| IBIS file was generated by Viper version: 2022.03.25
[IBIS Ver]   4.2
[Comment Char]   |_char
[File Name]   n9xx_150mhz_100hlqfp_14x14_p02g.ibs
[File Rev]   1.0
[Date]   Mon Apr  4 13:26:27 2022
[Source]   NXP Viper 2022.03.25
[Notes]
[Disclaimer] IMPORTANT NOTICE
  This information is provided on an AS IS basis and without warranty.
  IN NO EVENT SHALL NXP BE LIABLE FOR INCIDENTAL OR CONSEQUENTIAL
  DAMAGES ARISING FROM USE OF THIS INFORMATION. THIS DISCLAIMER OF
  WARRANTY EXTENDS TO THE USER OF THE INFORMATION, AND TO THEIR CUSTOMERS
  OR USERS OF PRODUCTS  AND IS IN LIEU OF ALL WARRANTIES WHETHER EXPRESS,
  IMPLIED, OR STATUTORY, INCLUDING IMPLIED WARRANTIES OF MERCHANTABILITY
  OR FITNESS FOR PARTICULAR PURPOSE.
  NXP does not represent or warrant that the information furnished
  hereunder is free of infringement of any third party patents,
  copyrights, trade secrets, or other intellectual property rights.
  NXP does not represent or warrant that the information is free of
  defect, or that it meets any particular standard, requirements or need
  of the user of the infomation or their customers.
  NXP reserves the right to change the information in this file
  without notice.
   http://www.nxp.com
[Copyright]   (C) Copyright NXP 2004 - 2022, All Rights Reserved.
|   MCXN_100HLQFP_14x14_N9XX
[Component]   MCXN_100HLQFP_14x14_N9XX
[Manufacturer]   NXP
[Package]
| variable   typ   min   max
R_pkg   0.23129   0.12177   0.27328
L_pkg   4.788e-09   3.815e-09   5.696e-09
C_pkg   3.794e-13   3.182e-13   7.043e-13
[Pin] signal_name   model_name   R_pin   L_pin   C_pin
1   P1_8   a_ip_io_3v_3p3v   0.25423   5.614e-09 4.032e-13
2   P1_9   a_ip_io_3v_3p3v   0.24672   5.246e-09 3.972e-13
3   P1_10   a_ip_io_3v_3p3v   0.24265   5.154e-09 3.883e-13
4   P1_11   a_ip_io_3v_3p3v   0.23836   5.083e-09 3.818e-13
5   P1_12   a_ip_io_3v_3p3v   0.23426   4.951e-09 3.769e-13
6   P1_13   a_ip_io_3v_3p3v   0.2353   4.835e-09 3.729e-13
7   P1_14   a_ip_io_3v_3p3v   0.2403   4.758e-09 3.682e-13
8   P1_15   a_ip_io_3v_3p3v   0.25157   4.669e-09 3.655e-13
9   RESET_B   a_ip_io_3v_3p3v   0.24167   4.709e-09 3.458e-13
10   P1_30   a_ip_io_3v_3p3v   0.2458   4.703e-09 3.510e-13
11   P1_31   a_ip_io_3v_3p3v   0.2572   4.600e-09 3.513e-13
12   VDD_CORE   POWER   NA   NA   NA
13   VDD   POWER   NA   NA   NA
14   P2_0   NC   0.27071   4.771e-09 3.447e-13
15   P2_1   a_ip_io_3v_3p3v   0.25126   4.722e-09 3.490e-13
16   P2_2   a_ip_io_3v_3p3v   0.24437   4.717e-09 3.546e-13
17   P2_3   a_ip_io_3v_3p3v   0.24352   4.712e-09 3.617e-13
18   P2_4   a_ip_io_3v_3p3v   0.24721   4.785e-09 3.684e-13
19   P2_5   a_ip_io_3v_3p3v   0.25684   4.768e-09 3.762e-13
20   P2_6   a_ip_io_3v_3p3v   0.25449   4.963e-09 3.790e-13
21   P2_7   a_ip_io_3v_3p3v   0.25831   5.064e-09 3.849e-13
22   P4_0   a_ip_io_3v_3p3v   0.15187   4.592e-09 4.366e-13
23   P4_1   a_ip_io_3v_3p3v   0.15584   4.720e-09 4.572e-13
24   P4_2   a_ip_io_3v_3p3v   0.24701   5.327e-09 4.019e-13
25   P4_3   a_ip_io_3v_3p3v   0.25004   5.370e-09 4.035e-13
26   P4_4   a_ip_io_3v_3p3v   0.16172   5.017e-09 4.680e-13
27   P4_5   a_ip_io_3v_3p3v   0.16022   4.810e-09 4.695e-13
28   P4_6   a_ip_io_3v_3p3v   0.16313   4.664e-09 4.591e-13
29   P4_7   a_ip_io_3v_3p3v   0.12458   4.127e-09 5.115e-13
30   VDD_ANA   POWER   NA   NA   NA
31   VREFH   POWER   0.14876   4.210e-09 4.282e-13
32   VREFL   GND   0.22491   4.419e-09 3.580e-13
33   VSS_P4   GND   NA   NA   NA
34   VDD_P4   POWER   NA   NA   NA
35   P4_12   a_ip_io_3v_3p3v   0.22844   4.359e-09 3.397e-13
36   P4_13   a_ip_io_3v_3p3v   0.14745   4.108e-09 3.875e-13
37   P4_15   a_ip_io_3v_3p3v   0.24012   4.708e-09 3.182e-13
38   P4_16   NC   0.24983   4.781e-09 3.254e-13
39   P4_17   a_ip_io_3v_3p3v   0.15737   4.280e-09 3.837e-13
40   P4_19   a_ip_io_3v_3p3v   0.23221   4.583e-09 3.317e-13
41   P4_20   a_ip_io_3v_3p3v   0.2327   4.602e-09 3.454e-13
42   P4_21   a_ip_io_3v_3p3v   0.146   4.143e-09 4.131e-13
43   P4_23   a_ip_io_3v_3p3v   0.23703   4.568e-09 3.483e-13
44   VDD_USB   POWER   NA   NA   NA
45   USB0_DM   NC   0.22284   4.369e-09 3.625e-13
46   USB0_DP   NC   0.23027   4.424e-09 3.739e-13
47   VDD_BAT   POWER   NA   NA   NA
48   P5_0   a_ip_io_3v_1p8v   0.23912   4.867e-09 3.839e-13
49   P5_1   a_ip_io_3v_1p8v   0.23955   5.024e-09 3.974e-13
50   P5_2   a_ip_io_3v_1p8v   0.24843   5.356e-09 4.045e-13
51   P5_3   a_ip_io_3v_1p8v   0.24798   5.176e-09 3.979e-13
52   VSS_DCDC   GND   NA   NA   NA
53   DCDC_LX   NC   0.12177   3.815e-09 7.043e-13
54   VDD_DCDC   POWER   NA   NA   NA
55   VDD_SYS   POWER   NA   NA   NA
56   P3_21   a_ip_io_3v_1p8v   0.26939   4.870e-09 3.973e-13
57   P3_20   a_ip_io_3v_1p8v   0.26266   4.731e-09 3.853e-13
58   VDD_CORE   POWER   NA   NA   NA
59   VDD_P3   POWER   NA   NA   NA
60   P3_17   a_ip_io_3v_1p8v   0.26691   4.809e-09 3.713e-13
61   P3_16   a_ip_io_3v_1p8v   0.26293   4.844e-09 3.649e-13
62   P3_15   a_ip_io_3v_1p8v   0.26865   4.990e-09 3.514e-13
63   P3_14   a_ip_io_3v_1p8v   0.27328   5.070e-09 3.477e-13
64   P3_13   a_ip_io_3v_1p8v   0.26472   4.956e-09 3.441e-13
65   P3_12   a_ip_io_3v_1p8v   0.25587   4.669e-09 3.484e-13
66   VDD_P3   POWER   NA   NA   NA
67   P3_11   a_ip_io_3v_1p8v   0.24302   4.496e-09 3.614e-13
68   P3_10   a_ip_io_3v_1p8v   0.23776   4.655e-09 3.630e-13
69   P3_9   a_ip_io_3v_1p8v   0.23969   4.796e-09 3.688e-13
70   P3_8   a_ip_io_3v_1p8v   0.242   4.857e-09 3.786e-13
71   P3_7   a_ip_io_3v_1p8v   0.24897   4.983e-09 3.880e-13
72   P3_6   a_ip_io_3v_1p8v   0.26422   4.985e-09 4.023e-13
73   VDD_P3   POWER   NA   NA   NA
74   P3_1   a_ip_io_3v_1p8v   0.25078   5.206e-09 3.982e-13
75   P3_0   a_ip_io_3v_1p8v   0.25659   5.400e-09 4.078e-13
76   P0_0   a_ip_io_3v_3p3v   0.26287   5.696e-09 4.116e-13
77   P0_1   a_ip_io_3v_3p3v   0.25446   5.469e-09 4.061e-13
78   P0_2   a_ip_io_3v_3p3v   0.23999   5.036e-09 3.921e-13
79   P0_3   a_ip_io_3v_3p3v   0.22875   4.809e-09 3.803e-13
80   P0_4   a_ip_io_3v_3p3v   0.22017   4.637e-09 3.693e-13
81   P0_5   a_ip_io_3v_3p3v   0.21763   4.557e-09 3.590e-13
82   P0_6   a_ip_io_3v_3p3v   0.21829   4.539e-09 3.430e-13
83   VDD   POWER   NA   NA   NA
84   P0_16   a_ip_io_3v_3p3v   0.23726   4.587e-09 3.470e-13
85   P0_17   a_ip_io_3v_3p3v   0.23427   4.622e-09 3.441e-13
86   P0_18   a_ip_io_3v_3p3v   0.23551   4.675e-09 3.359e-13
87   P0_19   a_ip_io_3v_3p3v   0.24397   4.807e-09 3.254e-13
88   P0_20   a_ip_io_3v_3p3v   0.25138   4.901e-09 3.222e-13
89   P0_21   a_ip_io_3v_3p3v   0.24426   4.870e-09 3.218e-13
90   P0_22   a_ip_io_3v_3p3v   0.23502   4.662e-09 3.318e-13
91   P0_23   a_ip_io_3v_3p3v   0.2362   4.512e-09 3.360e-13
92   P1_0   a_ip_io_3v_3p3v   0.22164   4.521e-09 3.323e-13
93   P1_1   a_ip_io_3v_3p3v   0.21839   4.499e-09 3.437e-13
94   P1_2   a_ip_io_3v_3p3v   0.22062   4.551e-09 3.502e-13
95   P1_3   a_ip_io_3v_3p3v   0.22417   4.511e-09 3.610e-13
96   VDD   POWER   NA   NA   NA
97   P1_4   a_ip_io_3v_3p3v   0.2327   4.698e-09 3.737e-13
98   P1_5   a_ip_io_3v_3p3v   0.23692   5.056e-09 3.809e-13
99   P1_6   a_ip_io_3v_3p3v   0.23798   5.153e-09 3.940e-13
100   P1_7   a_ip_io_3v_3p3v   0.24452   5.277e-09 3.999e-13
101   VSS   GND   NA   NA   NA
[Pin Mapping]   pulldown_ref   pullup_ref
1   NC   NC
2   NC   NC
3   NC   NC
4   NC   NC
5   NC   NC
6   NC   NC
7   NC   NC
8   NC   NC
9   NC   NC
10   NC   NC
11   NC   NC
12   NC   VDD_CORE
13   NC   VDD
14   NC   NC
15   NC   NC
16   NC   NC
17   NC   NC
18   NC   NC
19   NC   NC
20   NC   NC
21   NC   NC
22   NC   NC
23   NC   NC
24   NC   NC
25   NC   NC
26   NC   NC
27   NC   NC
28   NC   NC
29   NC   NC
30   NC   VDD_ANA
31   NC   VREFH
32   VREFL   NC
33   VSS_P4   NC
34   NC   VDD_P4
35   NC   NC
36   NC   NC
37   NC   NC
38   NC   NC
39   NC   NC
40   NC   NC
41   NC   NC
42   NC   NC
43   NC   NC
44   NC   VDD_USB
45   NC   NC
46   NC   NC
47   NC   VDD_BAT
48   NC   NC
49   NC   NC
50   NC   NC
51   NC   NC
52   VSS_DCDC   NC
53   NC   NC
54   NC   VDD_DCDC
55   NC   VDD_SYS
56   NC   NC
57   NC   NC
58   NC   VDD_CORE
59   NC   VDD_P3
60   NC   NC
61   NC   NC
62   NC   NC
63   NC   NC
64   NC   NC
65   NC   NC
66   NC   VDD_P3
67   NC   NC
68   NC   NC
69   NC   NC
70   NC   NC
71   NC   NC
72   NC   NC
73   NC   VDD_P3
74   NC   NC
75   NC   NC
76   NC   NC
77   NC   NC
78   NC   NC
79   NC   NC
80   NC   NC
81   NC   NC
82   NC   NC
83   NC   VDD
84   NC   NC
85   NC   NC
86   NC   NC
87   NC   NC
88   NC   NC
89   NC   NC
90   NC   NC
91   NC   NC
92   NC   NC
93   NC   NC
94   NC   NC
95   NC   NC
96   NC   VDD
97   NC   NC
98   NC   NC
99   NC   NC
100   NC   NC
101   VSS   NC
|*   Model Selector   *
[Model Selector] a_ip_io_3v_1p8v
p_io_25mhz_ds0_sr0_1p8v_mio   dse=0 sre=0 25mhz
p_io_25mhz_ds0_sr1_1p8v_mio   dse=0 sre=1 25mhz
p_io_25mhz_ds1_sr0_1p8v_mio   dse=1 sre=0 25mhz
p_io_25mhz_ds1_sr1_1p8v_mio   dse=1 sre=1 25mhz
p_io_25mhz_r40_ds0_sr0_1p8v_mio   dse=0 sre=0 25mhz_r40
p_io_25mhz_r40_ds0_sr1_1p8v_mio   dse=0 sre=1 25mhz_r40
p_io_25mhz_r40_ds1_sr0_1p8v_mio   dse=1 sre=0 25mhz_r40
p_io_25mhz_r40_ds1_sr1_1p8v_mio   dse=1 sre=1 25mhz_r40
p_io_50mhz_ds0_sr0_1p8v_mio   dse=0 sre=0 50mhz
p_io_50mhz_ds0_sr1_1p8v_mio   dse=0 sre=1 50mhz
p_io_50mhz_ds1_sr0_1p8v_mio   dse=1 sre=0 50mhz
p_io_50mhz_ds1_sr1_1p8v_mio   dse=1 sre=1 50mhz
p_io_25mhz_cap_ds0_sr0_1p8v_mio   dse=0 sre=0 25mhz_cap
p_io_25mhz_cap_ds0_sr1_1p8v_mio   dse=0 sre=1 25mhz_cap
p_io_25mhz_cap_ds1_sr0_1p8v_mio   dse=1 sre=0 25mhz_cap
p_io_25mhz_cap_ds1_sr1_1p8v_mio   dse=1 sre=1 25mhz_cap
p_io_25mhz_2mux_ds0_sr0_1p8v_mio   dse=0 sre=0 25mhz_2mux
p_io_25mhz_2mux_ds0_sr1_1p8v_mio   dse=0 sre=1 25mhz_2mux
p_io_25mhz_2mux_ds1_sr0_1p8v_mio   dse=1 sre=0 25mhz_2mux
p_io_25mhz_2mux_ds1_sr1_1p8v_mio   dse=1 sre=1 25mhz_2mux
p_io_100mhz_ds0_sr0_1p8v_mio   dse=0 sre=0 100mhz
p_io_100mhz_ds0_sr1_1p8v_mio   dse=0 sre=1 100mhz
p_io_100mhz_ds1_sr0_1p8v_mio   dse=1 sre=0 100mhz
p_io_100mhz_ds1_sr1_1p8v_mio   dse=1 sre=1 100mhz
p_io_100mhz_weftd_ds0_sr0_1p8v_mio   dse=0 sre=0 100mhz
p_io_100mhz_weftd_ds0_sr1_1p8v_mio   dse=0 sre=1 100mhz
p_io_100mhz_weftd_ds1_sr0_1p8v_mio   dse=1 sre=0 100mhz
p_io_100mhz_weftd_ds1_sr1_1p8v_mio   dse=1 sre=1 100mhz
p_io_i2c_ds00_ds10_sr0_1p8v_mio   dse0=0 dse1=0 sre=0 i2c
p_io_i2c_ds00_ds10_sr1_1p8v_mio   dse0=0 dse1=0 sre=1 i2c
p_io_i2c_ds00_ds11_sr0_1p8v_mio   dse0=0 dse1=1 sre=0 i2c
p_io_i2c_ds00_ds11_sr1_1p8v_mio   dse0=0 dse1=1 sre=1 i2c
p_io_i2c_ds01_ds10_sr0_1p8v_mio   dse0=1 dse1=0 sre=0 i2c
p_io_i2c_ds01_ds10_sr1_1p8v_mio   dse0=1 dse1=0 sre=1 i2c
p_io_i2c_ds01_ds11_sr0_1p8v_mio   dse0=1 dse1=1 sre=0 i2c
p_io_i2c_ds01_ds11_sr1_1p8v_mio   dse0=1 dse1=1 sre=1 i2c
p_io_i2c_i2c1_1p8v_mio   ipp_i2c_lv=1 i2c
p_io_i2cfmp_ds00_ds10_sr0_1p8v_mio   dse0=0 dse1=0 sre=0 i2cfmp
p_io_i2cfmp_ds00_ds10_sr1_1p8v_mio   dse0=0 dse1=0 sre=1 i2cfmp
p_io_i2cfmp_ds00_ds11_sr0_1p8v_mio   dse0=0 dse1=1 sre=0 i2cfmp
p_io_i2cfmp_ds00_ds11_sr1_1p8v_mio   dse0=0 dse1=1 sre=1 i2cfmp
p_io_i2cfmp_ds01_ds10_sr0_1p8v_mio   dse0=1 dse1=0 sre=0 i2cfmp
p_io_i2cfmp_ds01_ds10_sr1_1p8v_mio   dse0=1 dse1=0 sre=1 i2cfmp
p_io_i2cfmp_ds01_ds11_sr0_1p8v_mio   dse0=1 dse1=1 sre=0 i2cfmp
p_io_i2cfmp_ds01_ds11_sr1_1p8v_mio   dse0=1 dse1=1 sre=1 i2cfmp
p_io_i2cfmp_i2c1_1p8v_mio   ipp_i2c_lv=1 i2cfmp
p_io_rst_1p8v_mio   rst
p_io_rst_rx1p8v_1p8v_mio   rst
p_io_aon_1p8v_mio   rst
[Model Selector] a_ip_io_3v_3p3v
p_io_25mhz_ds0_sr0_3p3v_mio   dse=0 sre=0 25mhz
p_io_25mhz_ds0_sr1_3p3v_mio   dse=0 sre=1 25mhz
p_io_25mhz_ds1_sr0_3p3v_mio   dse=1 sre=0 25mhz
p_io_25mhz_ds1_sr1_3p3v_mio   dse=1 sre=1 25mhz
p_io_25mhz_r40_ds0_sr0_3p3v_mio   dse=0 sre=0 25mhz_r40
p_io_25mhz_r40_ds0_sr1_3p3v_mio   dse=0 sre=1 25mhz_r40
p_io_25mhz_r40_ds1_sr0_3p3v_mio   dse=1 sre=0 25mhz_r40
p_io_25mhz_r40_ds1_sr1_3p3v_mio   dse=1 sre=1 25mhz_r40
p_io_50mhz_ds0_sr0_3p3v_mio   dse=0 sre=0 50mhz
p_io_50mhz_ds0_sr1_3p3v_mio   dse=0 sre=1 50mhz
p_io_50mhz_ds1_sr0_3p3v_mio   dse=1 sre=0 50mhz
p_io_50mhz_ds1_sr1_3p3v_mio   dse=1 sre=1 50mhz
p_io_25mhz_cap_ds0_sr0_3p3v_mio   dse=0 sre=0 25mhz_cap
p_io_25mhz_cap_ds0_sr1_3p3v_mio   dse=0 sre=1 25mhz_cap
p_io_25mhz_cap_ds1_sr0_3p3v_mio   dse=1 sre=0 25mhz_cap
p_io_25mhz_cap_ds1_sr1_3p3v_mio   dse=1 sre=1 25mhz_cap
p_io_25mhz_2mux_ds0_sr0_3p3v_mio   dse=0 sre=0 25mhz_2mux
p_io_25mhz_2mux_ds0_sr1_3p3v_mio   dse=0 sre=1 25mhz_2mux
p_io_25mhz_2mux_ds1_sr0_3p3v_mio   dse=1 sre=0 25mhz_2mux
p_io_25mhz_2mux_ds1_sr1_3p3v_mio   dse=1 sre=1 25mhz_2mux
p_io_100mhz_ds0_sr0_3p3v_mio   dse=0 sre=0 100mhz
p_io_100mhz_ds0_sr1_3p3v_mio   dse=0 sre=1 100mhz
p_io_100mhz_ds1_sr0_3p3v_mio   dse=1 sre=0 100mhz
p_io_100mhz_ds1_sr1_3p3v_mio   dse=1 sre=1 100mhz
p_io_100mhz_weftd_ds0_sr0_3p3v_mio   dse=0 sre=0 100mhz
p_io_100mhz_weftd_ds0_sr1_3p3v_mio   dse=0 sre=1 100mhz
p_io_100mhz_weftd_ds1_sr0_3p3v_mio   dse=1 sre=0 100mhz
p_io_100mhz_weftd_ds1_sr1_3p3v_mio   dse=1 sre=1 100mhz
p_io_i2c_ds00_ds10_sr0_3p3v_mio   dse0=0 dse1=0 sre=0 i2c
p_io_i2c_ds00_ds10_sr1_3p3v_mio   dse0=0 dse1=0 sre=1 i2c
p_io_i2c_ds00_ds11_sr0_3p3v_mio   dse0=0 dse1=1 sre=0 i2c
p_io_i2c_ds00_ds11_sr1_3p3v_mio   dse0=0 dse1=1 sre=1 i2c
p_io_i2c_ds01_ds10_sr0_3p3v_mio   dse0=1 dse1=0 sre=0 i2c
p_io_i2c_ds01_ds10_sr1_3p3v_mio   dse0=1 dse1=0 sre=1 i2c
p_io_i2c_ds01_ds11_sr0_3p3v_mio   dse0=1 dse1=1 sre=0 i2c
p_io_i2c_ds01_ds11_sr1_3p3v_mio   dse0=1 dse1=1 sre=1 i2c
p_io_i2c_i2c1_3p3v_mio   ipp_i2c_lv=1 i2c
p_io_i2cfmp_ds00_ds10_sr0_3p3v_mio   dse0=0 dse1=0 sre=0 i2cfmp
p_io_i2cfmp_ds00_ds10_sr1_3p3v_mio   dse0=0 dse1=0 sre=1 i2cfmp
p_io_i2cfmp_ds00_ds11_sr0_3p3v_mio   dse0=0 dse1=1 sre=0 i2cfmp
p_io_i2cfmp_ds00_ds11_sr1_3p3v_mio   dse0=0 dse1=1 sre=1 i2cfmp
p_io_i2cfmp_ds01_ds10_sr0_3p3v_mio   dse0=1 dse1=0 sre=0 i2cfmp
p_io_i2cfmp_ds01_ds10_sr1_3p3v_mio   dse0=1 dse1=0 sre=1 i2cfmp
p_io_i2cfmp_ds01_ds11_sr0_3p3v_mio   dse0=1 dse1=1 sre=0 i2cfmp
p_io_i2cfmp_ds01_ds11_sr1_3p3v_mio   dse0=1 dse1=1 sre=1 i2cfmp
p_io_i2cfmp_i2c1_3p3v_mio   ipp_i2c_lv=1 i2cfmp
p_io_rst_3p3v_mio   rst
p_io_rst_rx1p8v_3p3v_mio   rst
p_io_aon_3p3v_mio   rst
| End [Component] MCXN_100HLQFP_14x14_N9XX
| Models and submodels in the file (98): p_io_100mhz_ds0_sr0_1p8v_mio (I/O), p_io_100mhz_ds0_sr0_3p3v_mio (I/O), p_io_100mhz_ds0_sr1_1p8v_mio (I/O), p_io_100mhz_ds0_sr1_3p3v_mio (I/O), p_io_100mhz_ds1_sr0_1p8v_mio (I/O), p_io_100mhz_ds1_sr0_3p3v_mio (I/O), p_io_100mhz_ds1_sr1_1p8v_mio (I/O), p_io_100mhz_ds1_sr1_3p3v_mio (I/O), p_io_100mhz_weftd_ds0_sr0_1p8v_mio (I/O), p_io_100mhz_weftd_ds0_sr0_3p3v_mio (I/O), p_io_100mhz_weftd_ds0_sr1_1p8v_mio (I/O), p_io_100mhz_weftd_ds0_sr1_3p3v_mio (I/O), p_io_100mhz_weftd_ds1_sr0_1p8v_mio (I/O), p_io_100mhz_weftd_ds1_sr0_3p3v_mio (I/O), p_io_100mhz_weftd_ds1_sr1_1p8v_mio (I/O), p_io_100mhz_weftd_ds1_sr1_3p3v_mio (I/O), p_io_25mhz_2mux_ds0_sr0_1p8v_mio (I/O), p_io_25mhz_2mux_ds0_sr0_3p3v_mio (I/O), p_io_25mhz_2mux_ds0_sr1_1p8v_mio (I/O), p_io_25mhz_2mux_ds0_sr1_3p3v_mio (I/O), p_io_25mhz_2mux_ds1_sr0_1p8v_mio (I/O), p_io_25mhz_2mux_ds1_sr0_3p3v_mio (I/O), p_io_25mhz_2mux_ds1_sr1_1p8v_mio (I/O), p_io_25mhz_2mux_ds1_sr1_3p3v_mio (I/O), p_io_25mhz_cap_ds0_sr0_1p8v_mio (I/O), p_io_25mhz_cap_ds0_sr0_3p3v_mio (I/O), p_io_25mhz_cap_ds0_sr1_1p8v_mio (I/O), p_io_25mhz_cap_ds0_sr1_3p3v_mio (I/O), p_io_25mhz_cap_ds1_sr0_1p8v_mio (I/O), p_io_25mhz_cap_ds1_sr0_3p3v_mio (I/O), p_io_25mhz_cap_ds1_sr1_1p8v_mio (I/O), p_io_25mhz_cap_ds1_sr1_3p3v_mio (I/O), p_io_25mhz_ds0_sr0_1p8v_mio (I/O), p_io_25mhz_ds0_sr0_3p3v_mio (I/O), p_io_25mhz_ds0_sr1_1p8v_mio (I/O), p_io_25mhz_ds0_sr1_3p3v_mio (I/O), p_io_25mhz_ds1_sr0_1p8v_mio (I/O), p_io_25mhz_ds1_sr0_3p3v_mio (I/O), p_io_25mhz_ds1_sr1_1p8v_mio (I/O), p_io_25mhz_ds1_sr1_3p3v_mio (I/O), p_io_25mhz_r40_ds0_sr0_1p8v_mio (I/O), p_io_25mhz_r40_ds0_sr0_3p3v_mio (I/O), p_io_25mhz_r40_ds0_sr1_1p8v_mio (I/O), p_io_25mhz_r40_ds0_sr1_3p3v_mio (I/O), p_io_25mhz_r40_ds1_sr0_1p8v_mio (I/O), p_io_25mhz_r40_ds1_sr0_3p3v_mio (I/O), p_io_25mhz_r40_ds1_sr1_1p8v_mio (I/O), p_io_25mhz_r40_ds1_sr1_3p3v_mio (I/O), p_io_50mhz_ds0_sr0_1p8v_mio (I/O), p_io_50mhz_ds0_sr0_3p3v_mio (I/O), p_io_50mhz_ds0_sr1_1p8v_mio (I/O), p_io_50mhz_ds0_sr1_3p3v_mio (I/O), p_io_50mhz_ds1_sr0_1p8v_mio (I/O), p_io_50mhz_ds1_sr0_3p3v_mio (I/O), p_io_50mhz_ds1_sr1_1p8v_mio (I/O), p_io_50mhz_ds1_sr1_3p3v_mio (I/O), p_io_aon_1p8v_mio (I/O), p_io_aon_3p3v_mio (I/O), p_io_i2c_ds00_ds10_sr0_1p8v_mio (I/O), p_io_i2c_ds00_ds10_sr0_3p3v_mio (I/O), p_io_i2c_ds00_ds10_sr1_1p8v_mio (I/O), p_io_i2c_ds00_ds10_sr1_3p3v_mio (I/O), p_io_i2c_ds00_ds11_sr0_1p8v_mio (I/O), p_io_i2c_ds00_ds11_sr0_3p3v_mio (I/O), p_io_i2c_ds00_ds11_sr1_1p8v_mio (I/O), p_io_i2c_ds00_ds11_sr1_3p3v_mio (I/O), p_io_i2c_ds01_ds10_sr0_1p8v_mio (I/O), p_io_i2c_ds01_ds10_sr0_3p3v_mio (I/O), p_io_i2c_ds01_ds10_sr1_1p8v_mio (I/O), p_io_i2c_ds01_ds10_sr1_3p3v_mio (I/O), p_io_i2c_ds01_ds11_sr0_1p8v_mio (I/O), p_io_i2c_ds01_ds11_sr0_3p3v_mio (I/O), p_io_i2c_ds01_ds11_sr1_1p8v_mio (I/O), p_io_i2c_ds01_ds11_sr1_3p3v_mio (I/O), p_io_i2c_i2c1_1p8v_mio (I/O), p_io_i2c_i2c1_3p3v_mio (I/O), p_io_i2cfmp_ds00_ds10_sr0_1p8v_mio (I/O), p_io_i2cfmp_ds00_ds10_sr0_3p3v_mio (I/O), p_io_i2cfmp_ds00_ds10_sr1_1p8v_mio (I/O), p_io_i2cfmp_ds00_ds10_sr1_3p3v_mio (I/O)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
